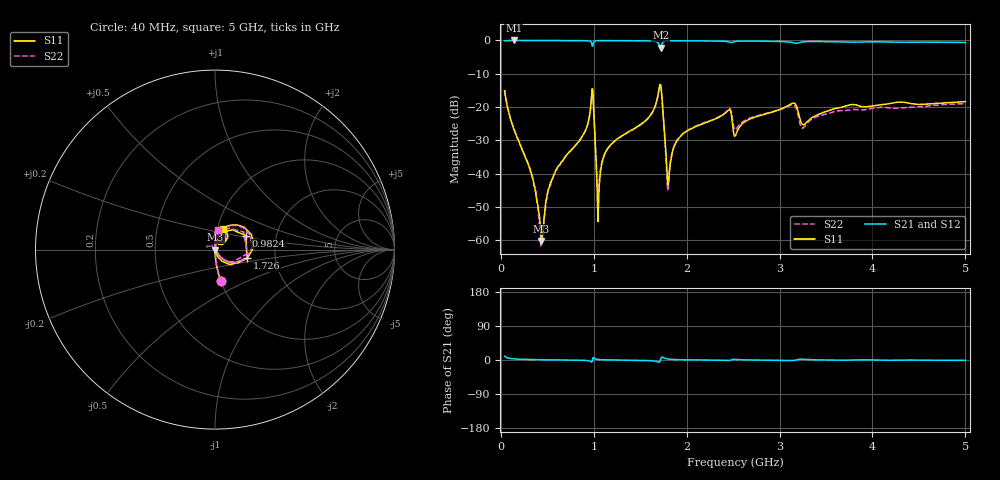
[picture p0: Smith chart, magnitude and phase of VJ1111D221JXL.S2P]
! VJ1111D221JXL
! DATE 02/15/2022  13:24
! CAPACITORS MOUNTED IN SERIES ON 25 MIL THICK MICROSTRIP SUBSTRATE
# GHz  S  MA  R  50.00
!  FREQ  S11M  S11A  S21M  S21A  S12M  S12A  S22M  S22A
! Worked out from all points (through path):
!   801 points, 40 MHz to 5 GHz, reference 50 ohm
!   highest |S21| = 0.00 dB at 139.2 MHz (marker M1); lowest = -2.1 dB at 1.72 GHz (marker M2)
!   lowest |S11| = -60.2 dB at 436.8 MHz (marker M3), VSWR 1.00, Z = 50.1 - j0.0295 ohm
!   |S11| at or under -10 dB: start of sweep to end of sweep
!   |S22| runs from -61.7 to -13.4 dB; largest |S21 - S12| = 0.01
!   S11 on the Smith chart (normalised r, x): 40 MHz: 1.00, -0.36; 982.4 MHz: 1.40, +0.22; 1.726 GHz: 1.43, -0.14; 5 GHz: 1.06, +0.24
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0.04  0.1768 -79.2  0.9843 10.1  0.9835 10.3  0.18 -79.4
0.1392  0.04627 -86.8  0.9996 3.0  0.9975 3.0  0.04818 -86.2
0.3562  0.006642 -80.6  0.9962 0.9  1.001 0.9  0.006814 -77.2
0.4368  0.0009803 -17.5  0.9951 0.6  1.001 0.6  0.0008525 -26.6
0.567  0.009329 81.7  0.9953 0.3  1 0.4  0.009297 85.9
0.8708  0.03565 82.9  0.9927 -0.7  0.9976 -0.7  0.03491 86.8
0.9824  0.1894 24.2  0.8305 -4.3  0.8367 -4.3  0.1872 31.5
1.032  0.008582 -65.6  0.9915 2.0  0.994 1.9  0.0102 -40.9
1.0568  0.005858 75.5  0.9939 1.2  0.9967 1.2  0.007611 58.1
1.1436  0.02316 86.9  0.9939 0.4  0.997 0.3  0.02329 85.4
1.6954  0.1638 56.7  0.9081 -5.7  0.9124 -5.8  0.1597 56.7
1.7202  0.215 3.1  0.782 2.5  0.7854 2.4  0.2077 3.0
1.7264  0.1865 -15.2  0.8205 6.6  0.825 6.4  0.1799 -15.5
1.8008  0.006778 25.4  0.9868 2.6  0.9912 2.5  0.006126 47.0
1.9868  0.04242 87.1  0.9876 0.6  0.9932 0.5  0.04294 89.2
2.4518  0.09052 64.5  0.9524 -1.3  0.9568 -1.4  0.0932 73.0
2.52  0.03666 63.8  0.9656 1.6  0.9719 1.5  0.0457 65.5
3.1338  0.1137 66.3  0.9332 -1.6  0.9379 -1.7  0.1086 69.9
3.2454  0.05505 56.6  0.9492 2.0  0.9539 1.9  0.04826 66.9
3.3508  0.07009 81.1  0.9659 0.8  0.9709 0.6  0.06678 90.0
4.1754  0.1124 75.0  0.9489 -0.6  0.9554 -0.8  0.09727 85.1
5  0.1208 69.7  0.9329 -1.0  0.9375 -1.3  0.1129 82.7
